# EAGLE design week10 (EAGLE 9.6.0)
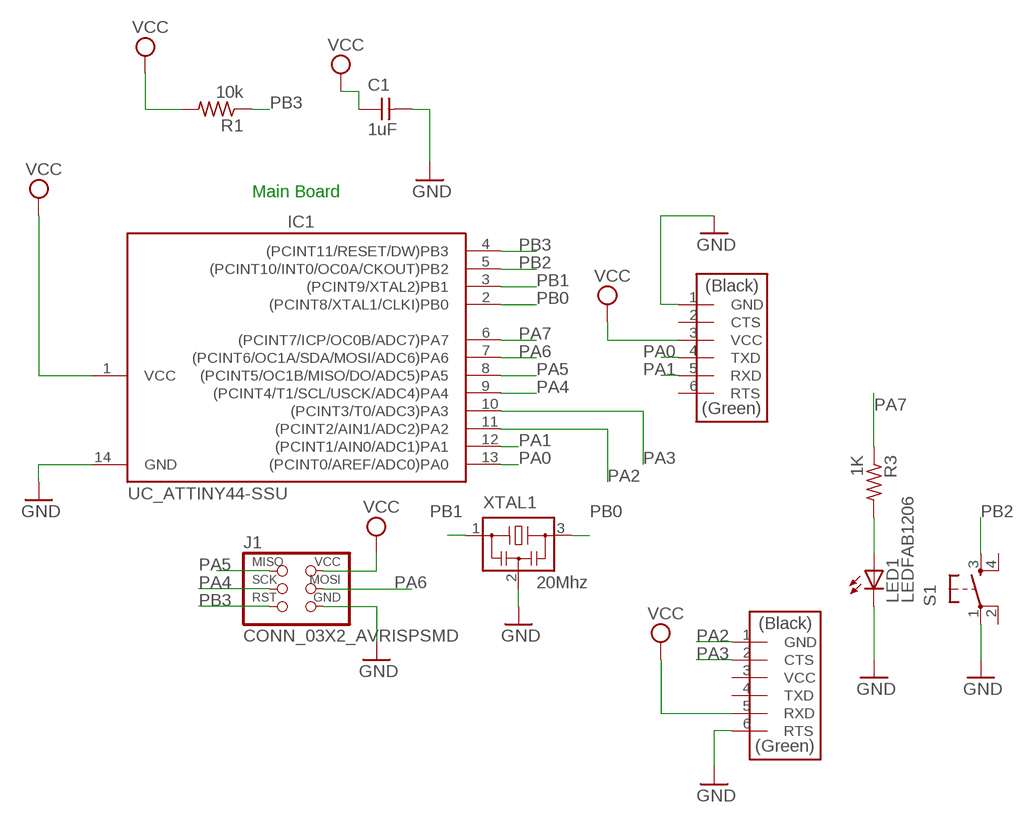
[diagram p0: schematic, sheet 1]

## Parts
C1  1uF  CAP_UNPOLARIZEDFAB  [C1206FAB]
IC1  UC_ATTINY44-SSU  [SOIC14]
J1  CONN_03X2_AVRISPSMD  [2X03SMD]
J2  CONN_06_FTDI-SMD-HEADER  [1X06SMD]
J3  CONN_06_FTDI-SMD-HEADER  [1X06SMD]
LED1  LEDFAB1206  [LED1206FAB]
R1  10k  R1206FAB  [R1206FAB]
R3  1K  R1206FAB  [R1206FAB]
S1  SW_SWITCH_TACTILE_6MM6MM_SWITCH  [6MM_SWITCH]
XTAL1  20Mhz  XTAL_RESONATOR  [EFOBM]

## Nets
GND: C1.2 IC1.14(GND) J1.6(GND) J2.1(GND) J3.6(RTS) LED1.2(C) S1.1(P) XTAL1.2
N$1: LED1.1(A) R3.2
PA0: IC1.13((PCINT0/AREF/ADC0)PA0) J2.4(TXD)
PA1: IC1.12((PCINT1/AIN0/ADC1)PA1) J2.5(RXD)
PA2: IC1.11((PCINT2/AIN1/ADC2)PA2) J3.1(GND)
PA3: IC1.10((PCINT3/T0/ADC3)PA3) J3.2(CTS)
PA4: IC1.9((PCINT4/T1/SCL/USCK/ADC4)PA4) J1.3(SCK)
PA5: IC1.8((PCINT5/OC1B/MISO/DO/ADC5)PA5) J1.1(MISO)
PA6: IC1.7((PCINT6/OC1A/SDA/MOSI/ADC6)PA6) J1.4(MOSI)
PA7: IC1.6((PCINT7/ICP/OC0B/ADC7)PA7) R3.1
PB0: IC1.2((PCINT8/XTAL1/CLKI)PB0) XTAL1.3
PB1: IC1.3((PCINT9/XTAL2)PB1) XTAL1.1
PB2: IC1.5((PCINT10/INT0/OC0A/CKOUT)PB2) S1.3(S)
PB3: IC1.4((PCINT11/RESET/DW)PB3) J1.5(RST) R1.1
VCC: C1.1 IC1.1(VCC) J1.2(VCC) J2.3(VCC) J3.5(RXD) R1.2
Unconnected: J2.2(CTS) J2.6(RTS) J3.3(VCC) J3.4(TXD) S1.2(P1) S1.4(S1)

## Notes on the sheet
- Main Board

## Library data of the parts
C1 = fab:CAP_UNPOLARIZED
IC1 = fab:UC_ATTINY44
J1 = fab:CONN_03X2_AVRISP
J2 J3 = fab:CONN_06_FTDI-SMD-HEADER
LED1 = fab:LED: LED
R1 R3 = fab:R: Resistor (US Symbol)
S1 = fab:SW_SWITCH_TACTILE_6MM: OMRON SWITCH
XTAL1 = fab:XTAL_RESONATOR

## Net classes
0 default: width 0.406 mm

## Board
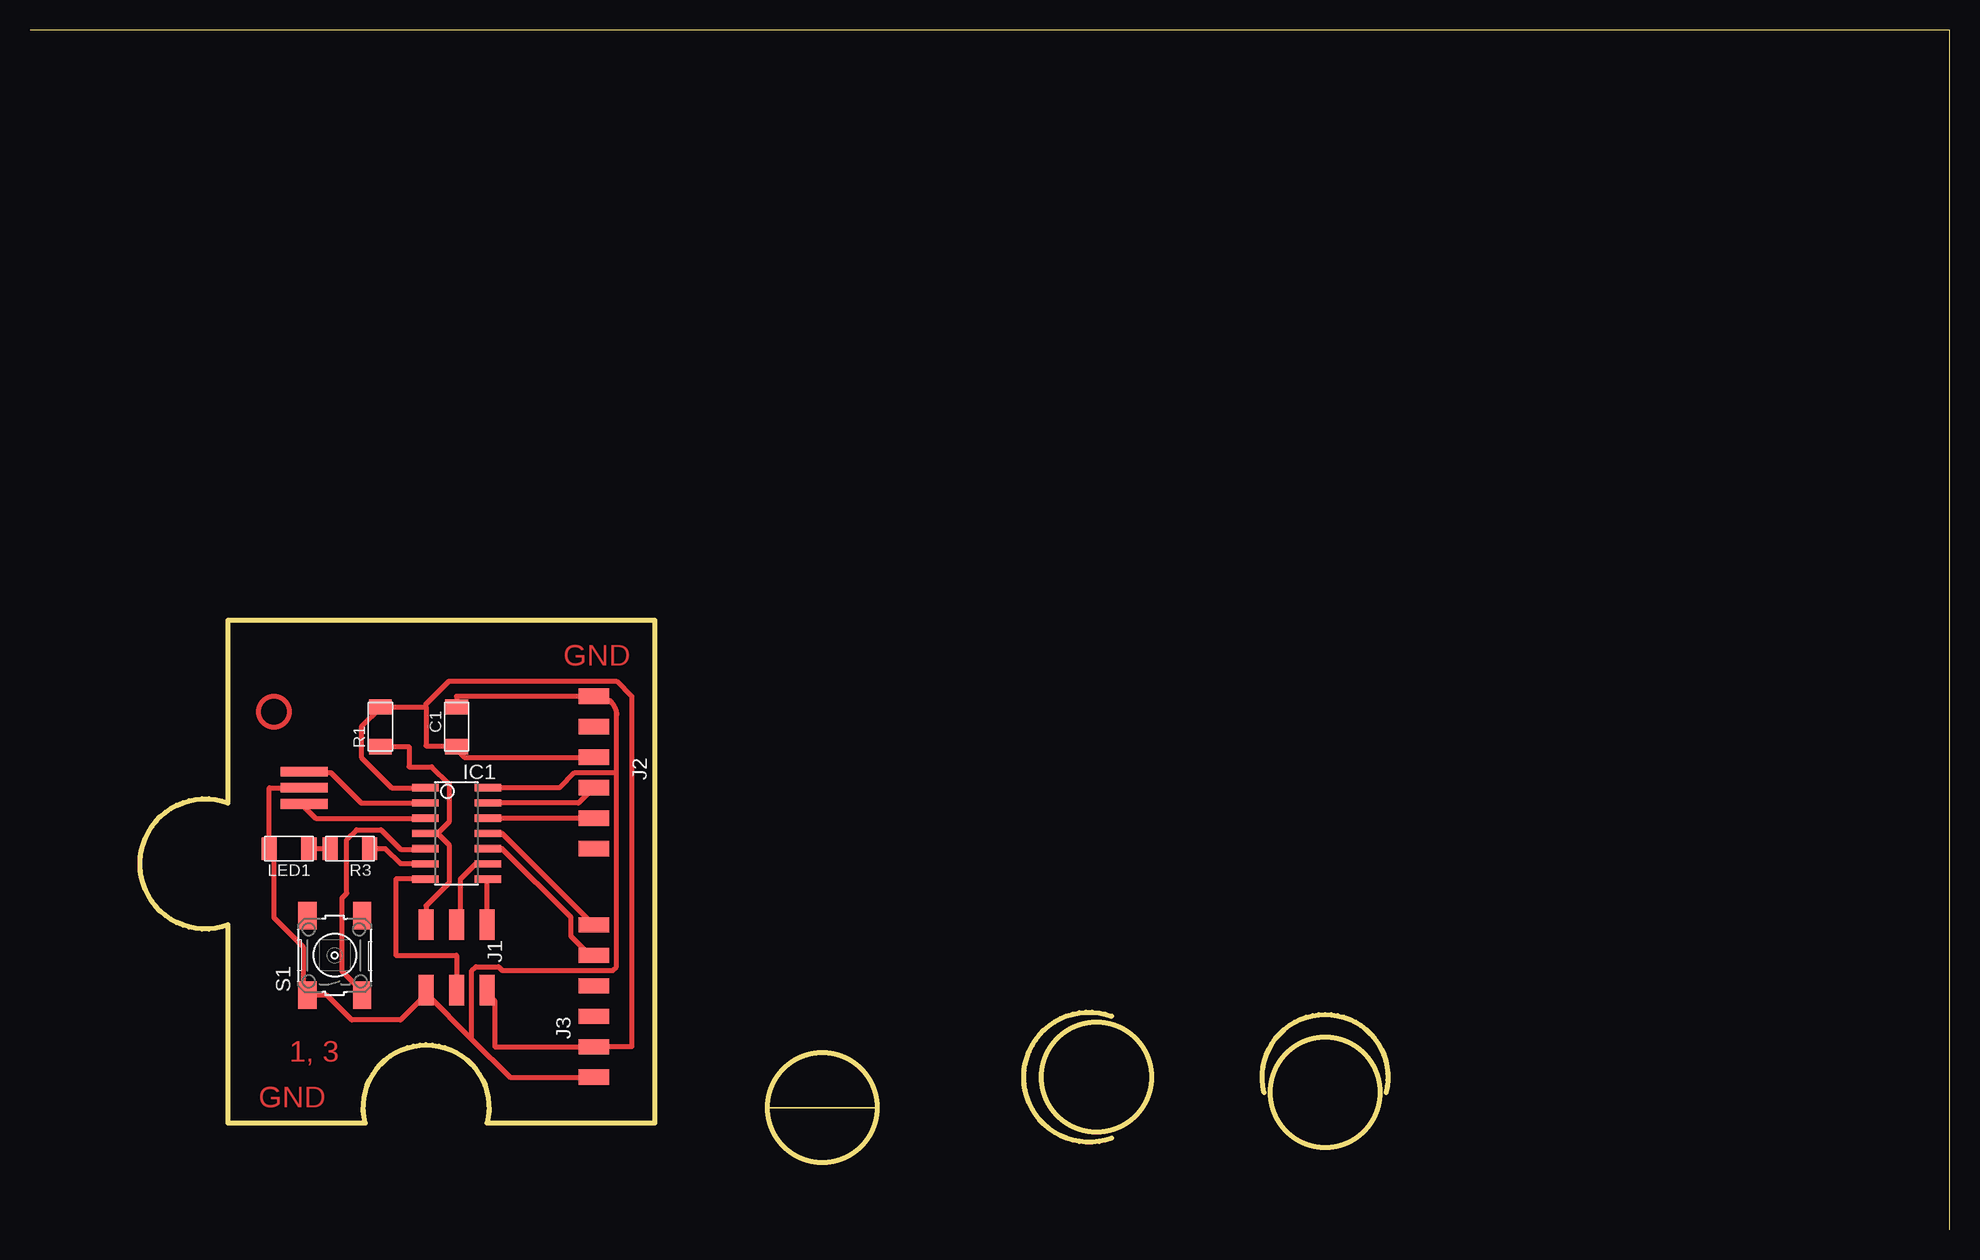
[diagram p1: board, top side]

Size 160 x 100 mm. Coordinates in mm from the lower left corner, seen from the top.
Outline: 160,0 160,100 0,100
Outline: 90.17,7.62 arc-221 90.17,17.78
Outline: 102.87,11.43 arc-208 113.03,11.43
Outline: 16.51,50.8 52.07,50.8 52.07,8.89 38.1,8.89 arc208 27.94,8.89 16.51,8.89 16.51,25.4 arc-221 16.51,35.56 16.51,50.8
Outline: circle at 66.04,10.16 radius 4.58
Outline: circle at 88.9,12.7 radius 4.58
Outline: circle at 107.95,11.43 radius 4.58
Copper layers (1*16): Top 0.035mm / dielectric 1.5mm / Bottom 0.035mm
Design rules "fab": minimum track width 10mil, minimum drill 32mil, track to track 16mil, track to pad 16mil, pad to pad 16mil, via to via 16mil, smd to smd 6mil, copper to edge 16mil, drill to drill 16mil, minimum pad ring 10mil, minimum via ring 8mil, stop-mask expansion 4mil, vias tented up to drill 0mil, thermal gap 16mil

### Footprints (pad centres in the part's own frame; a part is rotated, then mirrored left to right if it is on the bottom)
C1206FAB = smd 1.27 x 1.905: 1 -1.651,0; 2 1.651,0
SOIC14 = smd 0.61 x 2.21: 1 -3.81,-2.603; 2 -2.54,-2.603; 3 -1.27,-2.603; 4 0,-2.603; 5 1.27,-2.603; 6 2.54,-2.603; 7 3.81,-2.603; 8 3.81,2.603; 9 2.54,2.603; 10 1.27,2.603; 11 0,2.603; 12 -1.27,2.603; 13 -2.54,2.603; 14 -3.81,2.603
2X03SMD = smd 2.54 x 1.27: 1 -2.54,2.54; 2 2.92,2.54; 3 -2.54,0; 4 2.92,0; 5 -2.54,-2.54; 6 2.92,-2.54
1X06SMD = smd 2.54 x 1.27: 1 0,6.35; 2 0,3.81; 3 0,1.27; 4 0,-1.27; 5 0,-3.81; 6 0,-6.35
LED1206FAB = smd 1.27 x 1.905: 1 -1.651,0; 2 1.651,0
R1206FAB = smd 1.27 x 1.905: 1 -1.651,0; 2 1.651,0
6MM_SWITCH = smd 2.286 x 1.524: 1 -3.302,2.286; 2 3.302,2.286; 3 -3.302,-2.286; 4 3.302,-2.286
EFOBM = smd 0.8 x 3.9: 1 -1.35,0; 2 0,0; 3 1.35,0

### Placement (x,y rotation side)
C1  35.56,41.91 90 top
IC1  35.56,33.02 270 top
J1  35.56,22.86 270 top
J2  46.99,38.1 0 top
J3  46.99,19.05 0 top
LED1  21.59,31.75 180 top
R1  29.21,41.91 90 top
R3  26.67,31.75 180 top
S1  25.4,22.86 90 top
XTAL1  22.86,36.83 90 top

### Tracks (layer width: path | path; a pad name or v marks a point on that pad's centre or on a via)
GND
  Top 0.406: C1.2 35.56,44.45 J2.1 47.31,44.45 arc-90 48.9,42.86 48.9,38.1 | IC1.14 44.13,36.83 45.4,38.1 48.9,38.1 | XTAL1.2 19.94,36.83 LED1.2 20.32,31.7 20.32,26.01 22.76,23.57 22.76,19.91 S1.1 23.16,19.51 24.79,19.51 26.82,17.48 30.89,17.48 32.92,19.51 J1.6 33.02,19.68 36.83,15.88 | J3.6 40.01,12.7 36.83,15.88 | 48.9,38.1 48.9,21.91 48.58,21.59 39.37,21.59 39.05,21.91 37.15,21.91 36.83,21.59 36.83,15.88
N$1
  Top 0.406: R3.2 LED1.1
PA0
  Top 0.406: IC1.13 45.72,35.56 J2.4
PA1
  Top 0.406: J2.5 IC1.12
PA2
  Top 0.406: IC1.11 39.37,33.02 J3.1
PA3
  Top 0.406: IC1.10 39.37,31.75 45.09,26.04 45.09,24.45 46.67,22.86 J3.2
PA4
  Top 0.406: IC1.9 37.15,30.48 35.88,29.21 35.88,25.72 J1.3
PA5
  Top 0.406: J1.1 38.1,29.21 IC1.8
PA6
  Top 0.406: IC1.7 30.48,29.21 30.48,22.86 35.56,22.86 J1.4
PA7
  Top 0.406: IC1.6 30.89,30.48 29.62,31.75 R3.1
PB0
  Top 0.406: IC1.2 27.62,35.56 25.08,38.1 22.86,38.1 XTAL1.3
PB1
  Top 0.406: IC1.3 23.81,34.29 22.86,35.24 XTAL1.1
PB2
  Top 0.406: IC1.5 32.92,31.7 30.89,31.7 29.26,33.33 27.23,33.33 26.42,32.51 26.42,28.04 26.01,27.64 26.01,21.54 27.64,19.91 S1.3
PB3
  Top 0.406: J1.5 33.02,26.99 34.92,28.89 34.92,32.07 33.97,33.02 | 33.97,33.02 34.92,33.97 34.92,37.15 33.5,38.58 31.59,38.58 31.59,40.26 R1.1 | 33.97,33.02 IC1.4
VCC
  Top 0.406: J2.3 36.2,39.37 35.56,40.01 C1.1 35.56,40.32 33.02,40.32 33.02,43.56 | 33.02,43.56 R1.2 29.21,43.5 27.62,41.91 27.62,39.37 30.16,36.83 IC1.1 | J1.2 38.1,19.68 38.73,19.05 38.73,15.24 J3.5 50.16,15.24 50.16,44.45 48.9,45.72 34.92,45.72 33.02,43.81 33.02,43.56
(copper drawn outside any net)
  shapes: Top circle x1

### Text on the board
Top: GND | 1, 3 | GND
